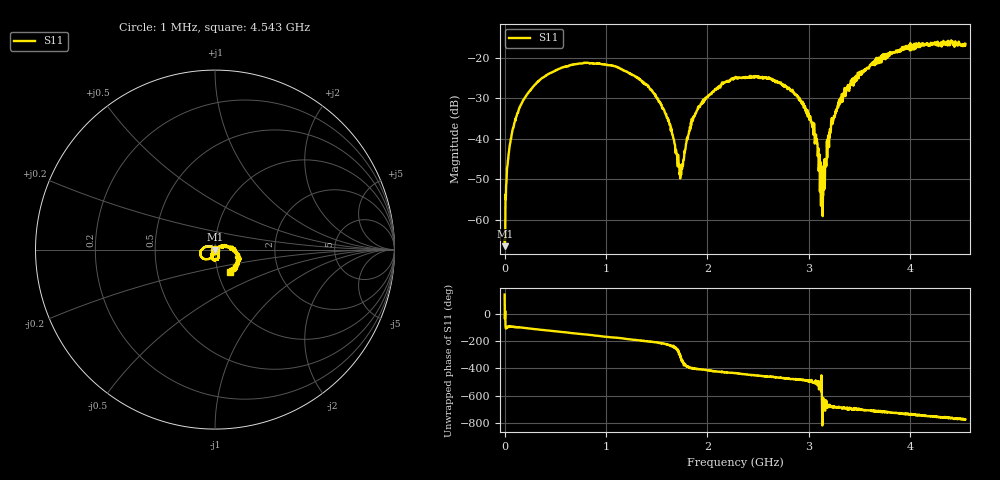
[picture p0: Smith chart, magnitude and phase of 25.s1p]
# HZ S RI R 50
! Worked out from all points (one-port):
!   1515 points, 1 MHz to 4.543 GHz, reference 50 ohm
!   lowest |S11| = -66.5 dB at 4 MHz (marker M1), VSWR 1.00, Z = 50 - j0.0296 ohm
!   |S11| at or under -10 dB: start of sweep to end of sweep
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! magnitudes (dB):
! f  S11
! 1 MHz  -65.0
! 4 MHz  -66.5
! 31 MHz  -46.3
! 46 MHz  -42.7
! 136 MHz  -33.2
! 316 MHz  -26.2
! 571 MHz  -22.4
! 1.138 GHz  -22.6
! 1.402 GHz  -26.6
! 1.528 GHz  -30.8
! 1.627 GHz  -36.6
! 1.705 GHz  -45.1
! 1.747 GHz  -46.3
! 1.831 GHz  -37.6
! 1.927 GHz  -32.0
! 2.272 GHz  -25.0
! 2.593 GHz  -25.0
! 2.842 GHz  -28.3
! 3.034 GHz  -37.1
! 3.085 GHz  -41.1
! 3.118 GHz  -56.4
! 3.13 GHz  -48.4
! 3.139 GHz  -53.8
! 3.229 GHz  -35.6
! 3.409 GHz  -26.4
! 3.724 GHz  -19.4
! 3.976 GHz  -17.7
! 4.543 GHz  -16.5
